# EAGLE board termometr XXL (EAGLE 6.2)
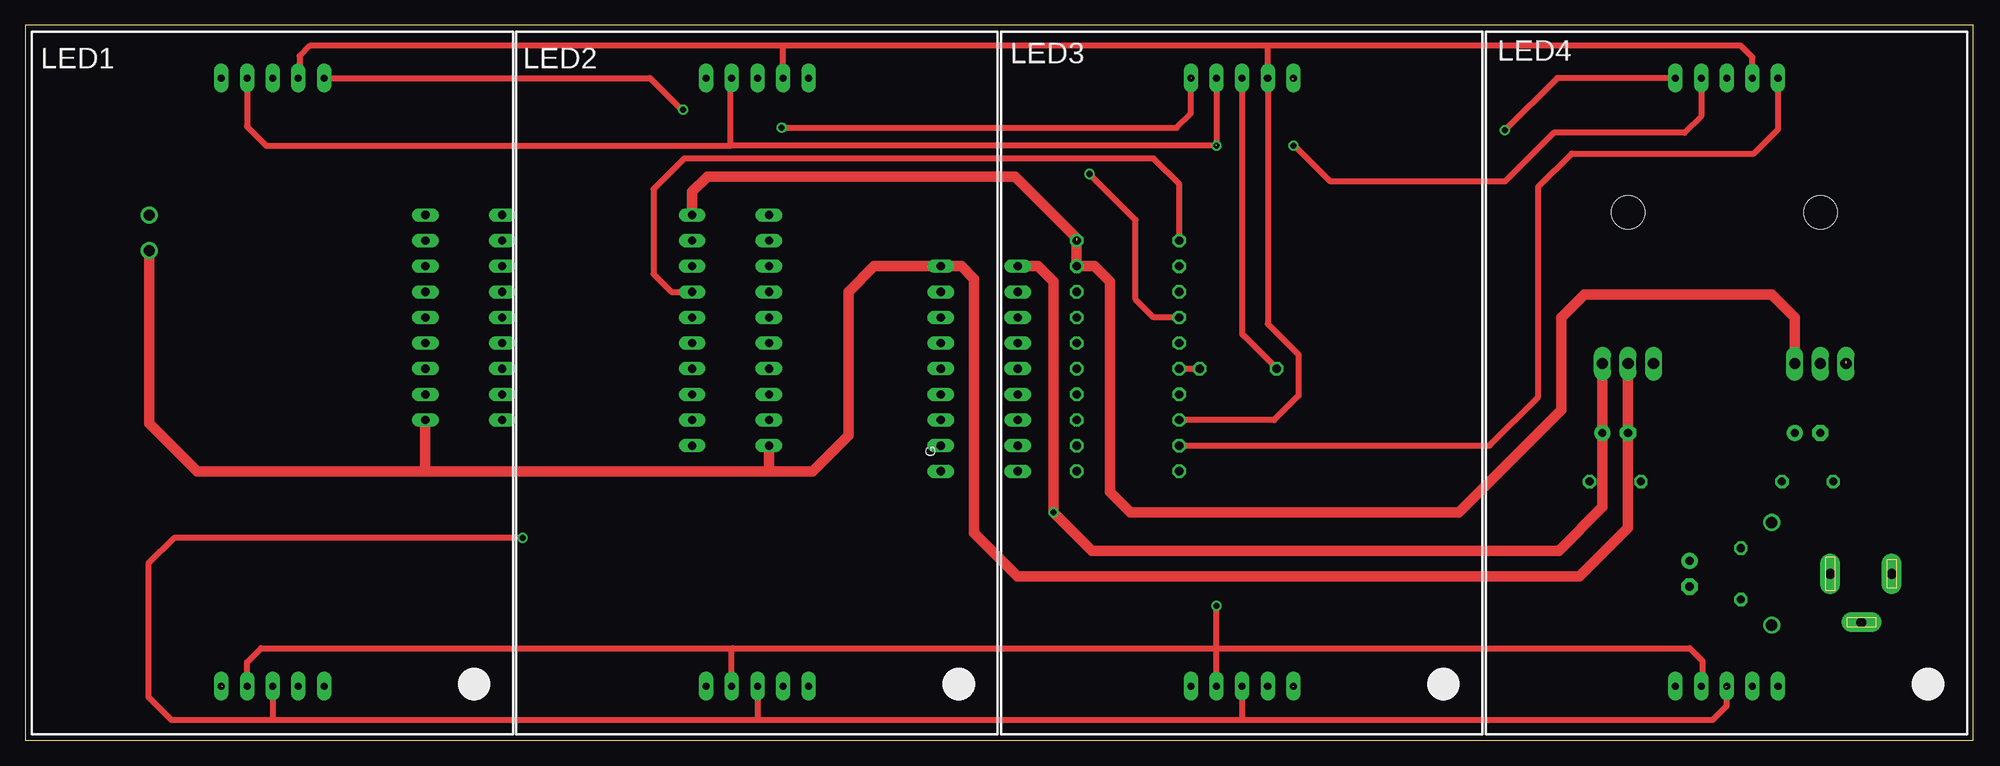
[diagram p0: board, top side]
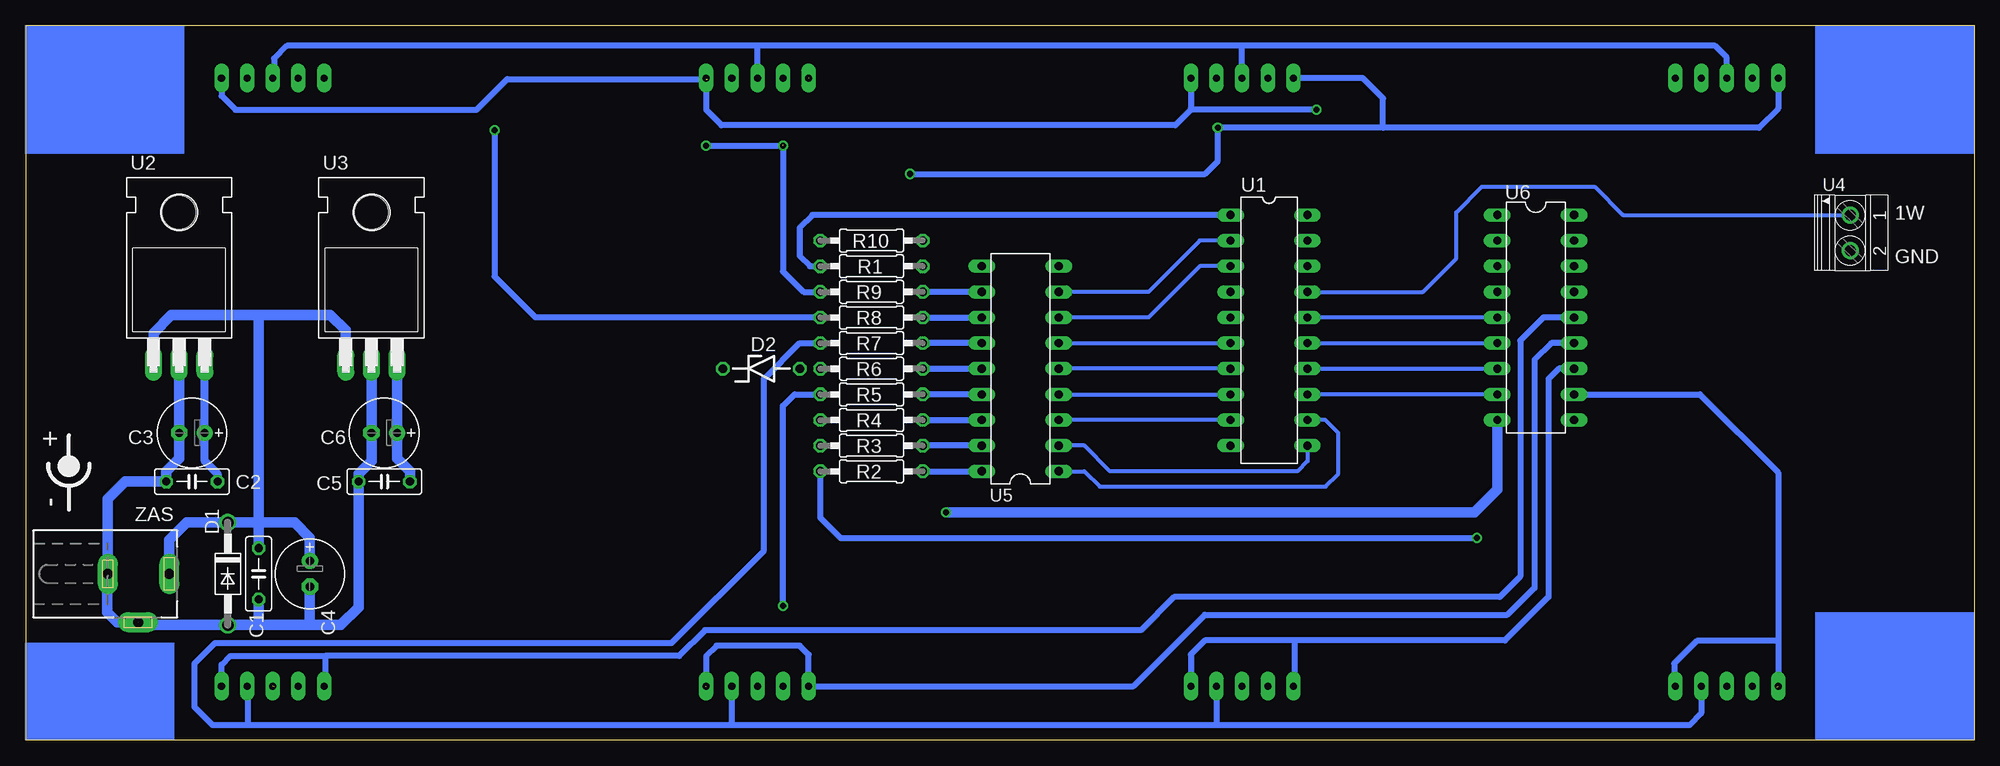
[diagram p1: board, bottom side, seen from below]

Size 192.96 x 70.86 mm. Coordinates in mm from the lower left corner, seen from the top.
Outline: 0,0 192.96,0 192.96,70.86 0,70.86 0,0
Copper layers (1*16): Top 0.035mm / dielectric 1.5mm / Bottom 0.035mm
Design rules: minimum track width 10mil, minimum drill 24mil, track to track 8mil, track to pad 8mil, pad to pad 8mil, via to via 8mil, smd to smd 8mil, copper to edge 40mil, drill to drill 8mil, minimum pad ring 10mil, minimum via ring 8mil, stop-mask expansion 4mil, vias tented up to drill 0mil, thermal gap 10mil

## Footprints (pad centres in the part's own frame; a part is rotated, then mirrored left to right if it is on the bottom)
C050-025X075 = drill 0.813 octagon: 1 -2.54,0; 2 2.54,0
E2,5-7 = drill 0.813 pad 1.6: + -1.27,0 | drill 0.813 pad 1.6 octagon: - 1.27,0
DO41-10 = drill 1.118: A 5.08,0; C -5.08,0
ZDIO-7.5 = drill 0.813 octagon: A 3.81,0; C -3.81,0
SA18-11 = drill 0.7 pad 1.422 long: 1 18.92,4.87; 2 21.46,4.87; 3 24,4.87; 4 26.54,4.87; 5 29.08,4.87; 6 18.92,65.13; 7 21.46,65.13; 8 24,65.13; 9 26.54,65.13; 10 29.08,65.13
0207/10 = drill 0.813 octagon: 1 -5.08,0; 2 5.08,0
DIL20 = drill 0.813 long: 1 -11.43,-3.81; 2 -8.89,-3.81; 3 -6.35,-3.81; 4 -3.81,-3.81; 5 -1.27,-3.81; 6 1.27,-3.81; 7 3.81,-3.81; 8 6.35,-3.81; 9 8.89,-3.81; 10 11.43,-3.81; 11 11.43,3.81; 12 8.89,3.81; 13 6.35,3.81; 14 3.81,3.81; 15 1.27,3.81; 16 -1.27,3.81; 17 -3.81,3.81; 18 -6.35,3.81; 19 -8.89,3.81; 20 -11.43,3.81
TO220H = drill 1.118 long: 1 -2.54,-10.16; 2 0,-10.16; 3 2.54,-10.16 | hole 3.302: 0,4.826
1751248 = drill 1.1 pad 1.7: 1 -1.75,-0.1; 2 1.75,-0.1
DIL18 = drill 0.813 long: 1 -10.16,-3.81; 2 -7.62,-3.81; 3 -5.08,-3.81; 4 -2.54,-3.81; 5 0,-3.81; 6 2.54,-3.81; 7 5.08,-3.81; 8 7.62,-3.81; 9 10.16,-3.81; 10 10.16,3.81; 11 7.62,3.81; 12 5.08,3.81; 13 2.54,3.81; 14 0,3.81; 15 -2.54,3.81; 16 -5.08,3.81; 17 -7.62,3.81; 18 -10.16,3.81
DCJ0202 = drill 1 pad 2 long: 1 0,3.1; 2 4.8,0; 3 0,-3

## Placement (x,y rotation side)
C1  100n  [C050-025X075]  169.93,16.51 90 bottom
C2  100n  [C050-025X075]  176.53,25.65 0 bottom
C3  100u  [E2,5-7]  176.53,30.48 180 bottom
C4  220u  [E2,5-7]  164.85,16.51 270 bottom
C5  100n  [C050-025X075]  157.48,25.65 0 bottom
C6  100u  [E2,5-7]  157.48,30.48 180 bottom
D1  1N4007  [DO41-10]  172.97,16.51 270 bottom
D2  5V1  [ZDIO-7.5]  120.14,36.83 0 bottom
LED1  7-SEG_SA18-11  [SA18-11]  0.51,0.51 0 top
LED2  7-SEG_SA18-11  [SA18-11]  48.51,0.51 0 top
LED3  7-SEG_SA18-11  [SA18-11]  96.52,0.51 0 top
LED4  7-SEG_SA18-11  [SA18-11]  144.53,0.51 0 top
R1  10k  [0207/10]  109.22,46.99 180 bottom
R2  [0207/10]  109.22,26.67 180 bottom
R3  [0207/10]  109.22,29.21 180 bottom
R4  [0207/10]  109.22,31.75 180 bottom
R5  [0207/10]  109.22,34.29 180 bottom
R6  [0207/10]  109.22,36.83 180 bottom
R7  [0207/10]  109.22,39.37 180 bottom
R8  [0207/10]  109.22,41.91 180 bottom
R9  [0207/10]  109.22,44.45 180 bottom
R10  10k  [0207/10]  109.22,49.53 180 bottom
U1  ATTINY2313  [DIL20]  69.85,40.64 270 bottom
U2  7805  [TO220H]  177.8,47.5 0 bottom
U3  7812  [TO220H]  158.75,47.5 0 bottom
U4  [1751248]  12.19,50.29 270 bottom
U5  ULN2803  [DIL18]  94.49,36.83 90 bottom
U6  UDN2983A  [DIL18]  43.43,41.91 270 bottom
ZAS  [DCJ0202]  181.86,16.51 270 bottom

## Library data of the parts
C1-C6 R1-R10 = rcl
D1 D2 = diode
LED1-LED4 = display-kingbright2; OC_FARNELL: unknown; OC_NEWARK: unknown
U1 = atmel; OC_FARNELL: unknown; OC_NEWARK: unknown
U2 U3 = linear
U4 = con-phoenix-350; OC_FARNELL: unknown; OC_NEWARK: unknown
U5 U6 = uln-udn
ZAS = con-jack; OC_FARNELL: unknown; OC_NEWARK: unknown

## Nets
1WIRE: R10.2 U1.17 U4.1
A: U1.2 U5.8
A1: U1.13 U6.8
A1`: LED1.1 LED1.5 U6.11
A2: U1.14 U6.7
A2`: LED2.1 LED2.5 U6.12
A3: U1.15 U6.6
A3`: LED3.1 LED3.5 U6.13
A4: U1.16 U6.5
A4`: LED4.1 LED4.5 U6.14
A`: LED1.7 LED2.7 LED3.7 LED4.7 R9.2
B: U1.3 U5.7
B`: LED1.6 LED2.6 LED3.6 LED4.6 R8.2
C: U1.6 U5.6
C`: LED1.4 LED2.4 LED3.4 LED4.4 R7.2
D: U1.12 U5.1
D`: LED1.3 LED2.3 LED3.3 LED4.3 R2.2
DP: U1.7 U5.5
DP`: D2.C LED1.8 LED2.8 LED3.8 LED4.8
E: U1.8 U5.4
E`: LED1.2 LED2.2 LED3.2 LED4.2 R5.2
F: U1.9 U5.3
F`: LED1.9 LED2.9 LED3.9 LED4.9 R4.2
G: U1.11 U5.2
G`: LED1.10 LED2.10 LED3.10 LED4.10 R3.2
GND: C1.1 C2.1 C3.- C4.- C5.1 C6.- D1.A U1.10 U2.2 U3.2 U4.2 U5.9 U6.10 ZAS.2 ZAS.3
N$1: R1.2 U1.1
N$2: R2.1 U5.18
N$3: R4.1 U5.16
N$4: D2.A R6.2
N$5: R5.1 U5.15
N$6: R6.1 U5.14
N$7: R7.1 U5.13
N$8: C1.2 C4.+ D1.C U2.1 U3.1 ZAS.1
N$9: R8.1 U5.12
N$10: R9.1 U5.11
N$11: R3.1 U5.17
V+: C5.2 C6.+ U3.3 U5.10 U6.9
VCC: C2.2 C3.+ R1.1 R10.1 U1.20 U2.3

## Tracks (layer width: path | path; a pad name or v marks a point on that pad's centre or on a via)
1WIRE
  Top 0.61: R10.2 114.3,55.12 111.76,57.66 65.28,57.66 62.23,54.61 62.23,46.23 64.01,44.45 U1.17
  Bottom 0.406: U1.17 54.61,44.45 51.31,47.75 51.31,52.32 48.77,54.86 37.59,54.86 34.8,52.07 12.32,52.07 U4.1
A
  Bottom 0.406: U1.2 76.71,49.53 81.79,44.45 U5.8
A1
  Bottom 0.406: U6.8 U1.13
A1`  (1 unrouted)
  Bottom 0.61: U6.11 27.18,34.29 19.43,26.54 19.43,9.87 | 19.43,9.87 19.43,5.59 | 19.3,5.33 19.3,5.08 19.56,5.33 | 19.56,5.33 19.43,5.59 | 19.43,5.59 19.3,5.33 | 19.3,5.33 19.56,5.33 | 19.43,9.87 27.47,9.87 29.72,7.62 29.72,5.51 LED1.5
A2
  Bottom 0.406: U1.14 U6.7
A2`
  Bottom 0.61: U6.12 41.15,36.83 42.16,35.81 42.16,14.22 46.48,9.91 67.31,9.91 | 67.31,9.91 76.2,9.91 77.6,8.51 77.6,6.14 LED2.5 | 67.31,9.91 67.31,5.5 LED2.1
A3
  Bottom 0.406: U1.15 U6.6
A3`  (1 unrouted)
  Bottom 0.61: U6.13 41.91,39.37 43.56,37.72 43.56,15.11 46.23,12.45 76.2,12.45 83.27,5.38 LED3.1 115.44,8.51 116.33,9.4 124.59,9.4 125.6,8.38 125.6,5.33 125.73,5.33
A4
  Bottom 0.406: U6.5 U1.16
A4`
  Bottom 0.61: U6.14 42.67,41.91 44.96,39.62 44.96,16.26 46.99,14.22 79.25,14.22 82.55,10.92 125.73,10.92 128.27,8.38 163.32,8.38 | LED4.1 163.32,5.5 163.32,8.13 163.32,8.38 | LED4.5 173.61,7.5 172.72,8.38 163.32,8.38
A`  (via drill 0.6)  (1 unrouted)
  Top 0.61: LED4.7 165.99,61.85 164.34,60.2 151.38,60.2 146.56,55.37 129.29,55.37 125.73,58.93 v125.6,58.93 | 69.85,58.93 69.85,65.51 LED2.7 | LED1.7 21.97,60.84 23.88,58.93 69.85,58.93 | LED3.7 117.98,59.05 | v117.98,58.93 69.85,58.93
  Bottom 0.61: v125.6,58.93 v117.98,58.93 117.98,46.48 115.95,44.45 R9.2
B
  Bottom 0.406: U1.3 76.71,46.99 81.79,41.91 U5.7
B`  (via drill 0.6)  (1 unrouted)
  Top 0.61: v74.93,60.71 114.05,60.71 115.44,62.1 115.44,65.66 | R8.2 111.76,41.91 109.98,43.69 109.98,51.56 v105.41,56.13 | LED4.6 151.74,65.64 v146.56,60.45
  Bottom 0.61: R8.2 142.49,41.91 146.56,45.97 v146.56,60.45 | LED1.6 19.43,62.61 21.34,60.71 58.55,60.71 | 58.55,60.71 58.55,63.63 60.55,65.64 LED2.6 | 58.55,60.71 v74.93,60.71 74.93,57.4 76.2,56.13 v105.41,56.13
C
  Bottom 0.406: U5.6 U1.6
C`
  Bottom 0.61: LED1.4 27.05,2.67 28.19,1.52 74.93,1.52 | 74.93,1.52 122.94,1.52 | 122.94,1.52 170.94,1.52 | 170.94,1.52 170.94,5.25 LED4.4 | LED3.4 123.06,1.65 122.94,1.52 | LED2.4 75.05,1.65 74.93,1.52 | 170.94,1.52 174.5,1.52 176.28,3.3 176.28,7.62 174.24,9.65 129.03,9.65 119.89,18.8 119.89,35.81 116.33,39.37 R7.2
D
  Bottom 0.406: U5.1 88.14,26.67 86.61,25.15 64.26,25.15 62.99,26.42 62.99,30.48 64.26,31.75 U1.12
D`  (via drill 0.6)  (1 unrouted)
  Top 0.61: v49.28,20.07 14.73,20.07 12.19,17.53 12.19,4.32 14.48,2.03 24.64,2.03 | 24.64,2.03 72.39,2.03 | 72.39,2.03 120.65,2.03 | 120.65,2.03 167.13,2.03 168.53,3.43 168.53,5.21 168.4,5.33 | LED1.3 24.51,2.16 24.64,2.03 | LED2.3 72.51,2.16 72.39,2.03 | LED3.3 120.52,2.16 120.65,2.03
  Bottom 0.61: R2.2 114.3,22.1 112.27,20.07 v49.28,20.07
DP
  Bottom 0.406: U1.7 U5.5
DP`
  Top 0.61: LED3.8 120.52,40.26 120.78,40 D2.C
  Bottom 0.61: LED1.8 24.51,67.69 25.65,68.83 72.39,68.83 | 72.39,68.83 120.4,68.83 | 120.4,68.83 167.13,68.83 168.4,67.56 168.4,65.76 LED4.8 | LED3.8 120.52,68.71 120.4,68.83 | LED2.8 72.51,68.71 72.39,68.83
E
  Bottom 0.406: U5.4 U1.8
E`  (via drill 0.6)
  Top 0.406: 166.12,5.51 LED4.2 | 117.98,8.77 117.98,9.14 | 69.97,9.01 70.1,9.14
  Top 0.61: LED1.2 21.97,7.74 23.37,9.14 70.1,9.14 117.98,9.14 | 117.98,9.14 164.85,9.14 166.12,7.87 166.12,5.51 | LED3.2 117.98,8.77 | LED2.2 69.97,9.01 | 117.98,9.14 v117.98,13.33
  Bottom 0.61: v117.98,13.33 117.98,33.15 116.84,34.29 R5.2
F
  Bottom 0.406: U1.9 U5.3
F`
  Top 0.61: LED4.9 171.07,67.69 169.93,68.83 123.19,68.83 | 123.19,68.83 74.93,68.83 | 74.93,68.83 28.19,68.83 27.18,67.82 27.18,65.77 LED1.9 | LED2.9 75.05,68.71 74.93,68.83 | 123.19,68.83 123.06,68.7 LED3.9 123.06,41.28 126.11,38.23 126.11,34.16 123.7,31.75 R4.2
G
  Bottom 0.406: U1.11 66.04,27.69 67.06,26.67 85.6,26.67 88.14,29.21 U5.2
G`  (via drill 0.6)  (1 unrouted)
  Top 0.61: R3.2 145.03,29.21 149.86,34.04 149.86,54.86 153.16,58.17 171.2,58.17 173.61,60.58 173.61,65.38 LED4.10 | LED1.10 61.87,65.64 65.02,62.48 v65.15,62.48
  Bottom 0.61: LED3.10 125.6,65.51 125.6,62.48 124.08,60.96 79.12,60.96 77.6,62.48 | LED4.10 173.61,63.88 172.21,62.48 148.34,62.48 145.29,65.53 125.48,65.53 | LED2.10 77.59,62.61 77.6,62.48 | v65.15,62.48 77.6,62.48
GND  (1 unrouted)
  Top 0.813: 39.62,26.92 39.88,26.67
  Top 1.016: 73.66,26.67 77.98,26.67 81.53,30.23 81.53,44.45 84.07,46.99 U5.9 92.71,46.99 93.98,45.72 93.98,20.57 98.3,16.26 153.92,16.26 158.75,21.08 U3.2 | 73.66,26.67 39.88,26.67 17.02,26.67 12.29,31.4 U4.2 | 73.66,26.67 U1.10 | U6.10 39.62,26.92
  Bottom 1.016: U3.2 C6.- 158.75,27.69 160.02,26.42 C5.1 160.02,13.21 161.8,11.43 164.59,11.43 | U2.2 C3.- 177.8,27.94 179.07,26.67 C2.1 183.13,25.65 184.86,23.92 ZAS.3 184.91,16.46 184.91,12.7 183.92,11.71 ZAS.2 | 164.59,11.43 169.93,11.43 | 169.93,11.43 D1.A 181.86,11.43 182.12,11.68 181.86,11.68 | C1.1 169.93,11.43 | C4.- 164.85,11.68 164.59,11.43
N$1
  Bottom 0.406: 114.55,46.99 R1.2
  Bottom 0.61: U1.1 115.06,52.07 116.33,50.8 116.33,48.01 115.32,46.99 114.55,46.99
N$2
  Bottom 0.61: R2.1 U5.18
N$3
  Bottom 0.61: R4.1 U5.16
N$4
  Top 0.61: R6.2 D2.A
N$5
  Bottom 0.61: U5.15 R5.1
N$6
  Bottom 0.61: R6.1 U5.14
N$7
  Bottom 0.61: U5.13 R7.1
N$8  (1 unrouted)
  Bottom 0.813: 180.34,37.59 180.59,37.34
  Bottom 1.016: U3.1 161.29,40.64 162.81,42.16 169.93,42.16 | 169.93,42.16 178.56,42.16 180.34,40.39 180.34,37.59 | 169.93,21.59 D1.C 177.04,21.59 178.76,19.86 ZAS.1 | 169.93,21.59 166.37,21.59 164.85,20.07 C4.+ | C1.2 169.93,21.59 | 169.93,21.59 169.93,42.16
N$9
  Bottom 0.61: R8.1 U5.12
N$10
  Bottom 0.61: U5.11 R9.1
N$11
  Bottom 0.61: U5.17 R3.1
V+  (via drill 0.6)
  Top 1.016: U5.10 100.33,46.99 101.85,45.47 v101.85,22.61 105.66,18.8 151.89,18.8 156.21,23.11 U3.3
  Bottom 1.016: C5.2 154.94,26.67 156.21,27.94 C6.+ U3.3 | U6.9 47.24,24.89 49.53,22.61 v101.85,22.61
VCC  (1 unrouted)
  Top 1.016: U1.20 66.04,54.36 67.56,55.88 98.04,55.88 104.14,49.78 R1.1 105.92,46.99 107.44,45.47 107.44,24.64 109.47,22.61 141.99,22.61 152.15,32.77 152.15,41.91 154.43,44.2 172.97,44.2 175.26,41.91 U2.3
  Bottom 0.813: U2.3 C3.+ 175.26,27.69 173.99,26.42 C2.2
(copper drawn outside any net)
  shapes: Bottom area x4

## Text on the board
tNames: G
bNames: 1W | GND | + | -
tStop: mosi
